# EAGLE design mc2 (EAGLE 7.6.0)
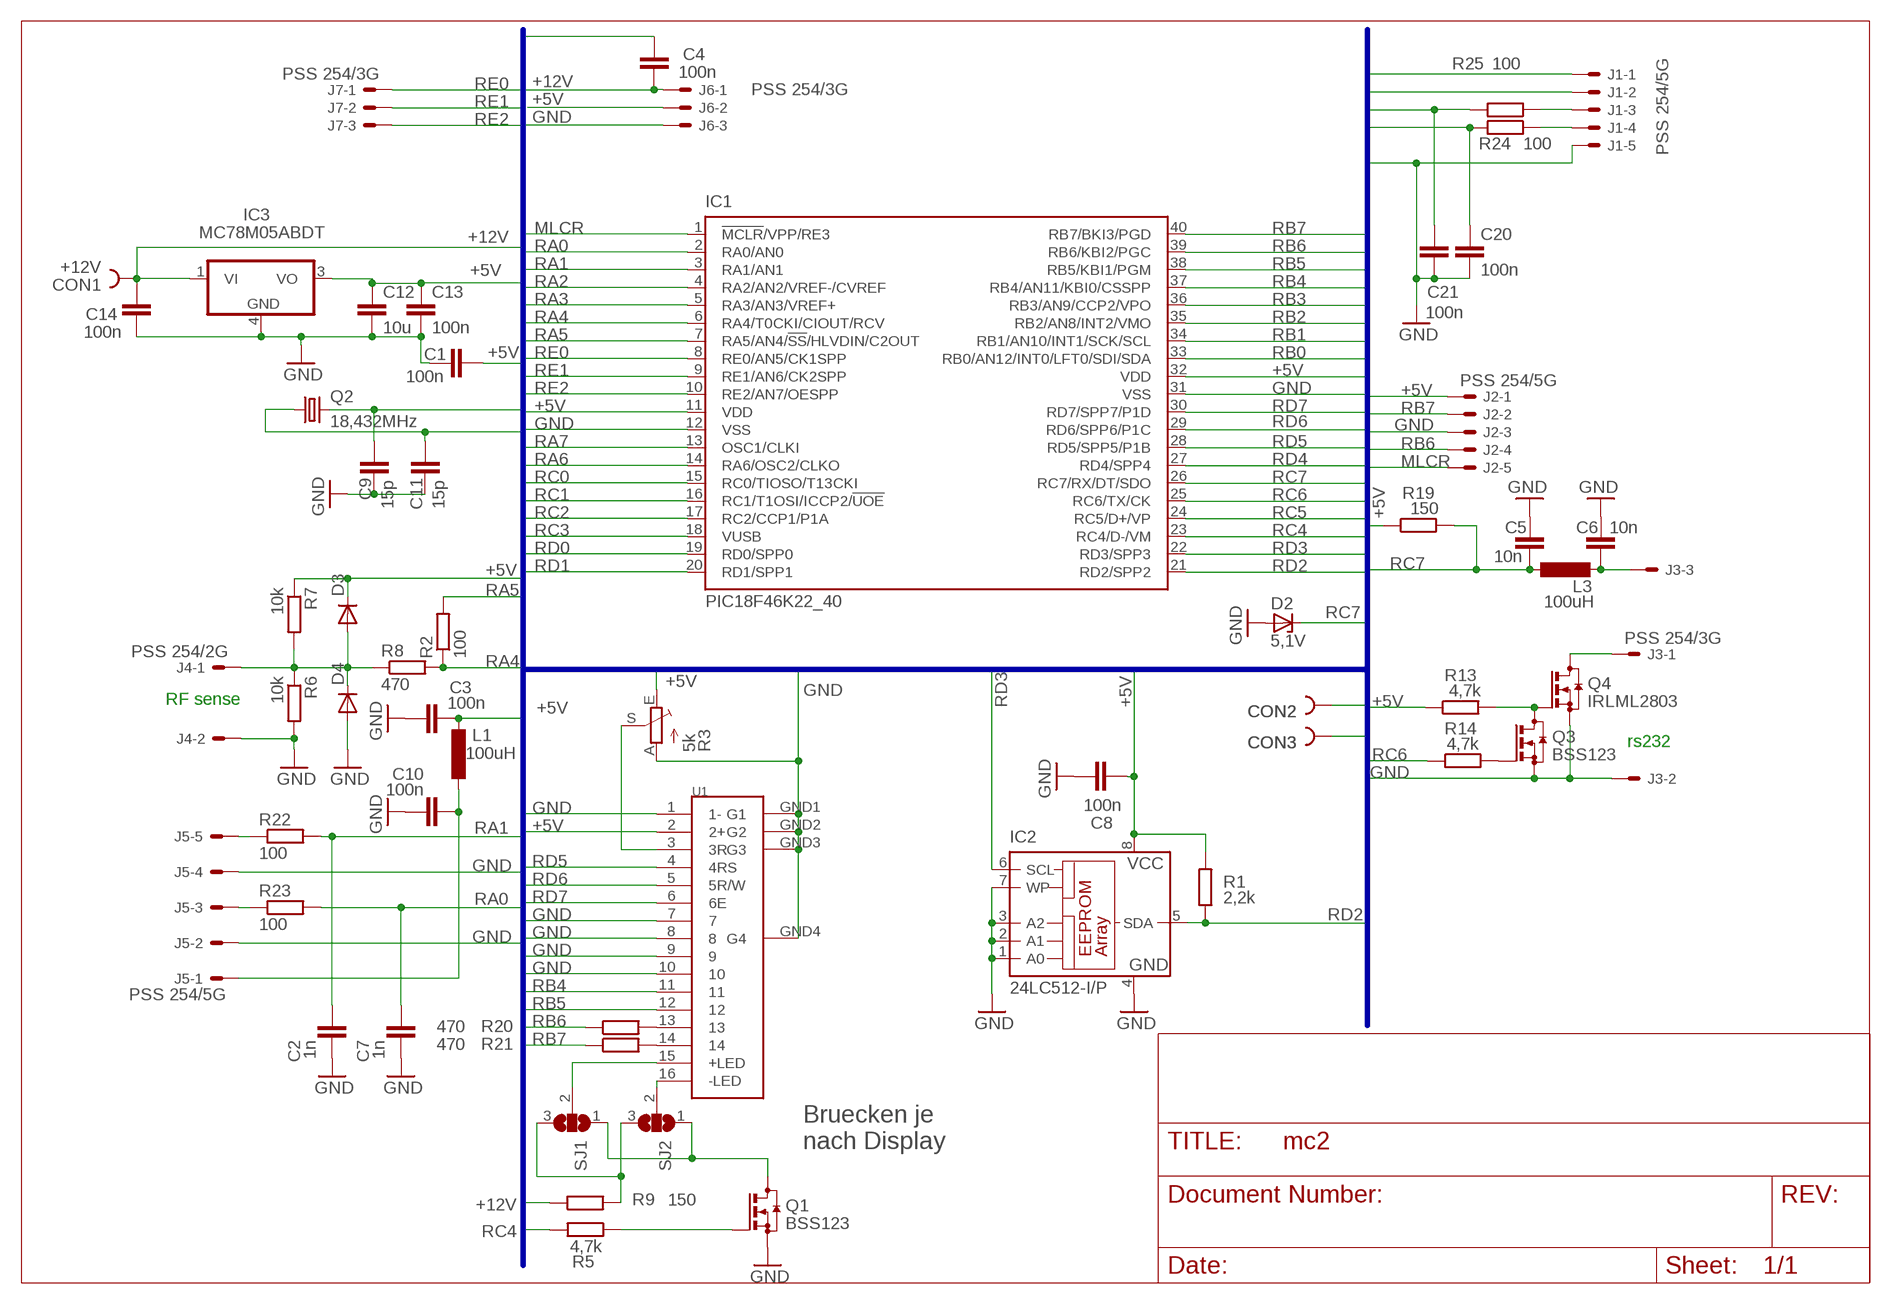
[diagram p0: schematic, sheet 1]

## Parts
C1  100n  C-EUC0805  [C0805]
C2  1n  C-EUC0805  [C0805]
C3  100n  C-EUC0805  [C0805]
C4  100n  C-EUC0805  [C0805]
C5  10n  C-EUC0805  [C0805]
C6  10n  C-EUC0805  [C0805]
C7  1n  C-EUC0805  [C0805]
C8  100n  C-EUC0805  [C0805]
C9  15p  C-EUC0805  [C0805]
C10  100n  C-EUC0805  [C0805]
C11  15p  C-EUC0805  [C0805]
C12  10u  C-EUC1206K  [C1206K]
C13  100n  C-EUC0805  [C0805]
C14  100n  C-EUC0805  [C0805]
C20  100n  C-EUC0805  [C0805]
C21  100n  C-EUC0805  [C0805]
CON1  +12V  PIN2_5  [PIN2_5]
CON2  PIN2_53MM  [HOLE3]
CON3  PIN2_53MM  [HOLE3]
D2  5,1V  ZENER-DIODESOT23  [SOT23]
D3  DIODE-SOD323-W  [SOD323-W]
D4  DIODE-SOD323-W  [SOD323-W]
IC1  PIC18F46K22_40  PIC18F4550_40  [DIL40]
IC2  24LC512-I/P  24AA32AP  [DIL8]
IC3  MC78M05ABDT  [DPACK_3]
J1  PSS 254/5G  22-27-2051-05  [6410-05]
J2  PSS 254/5G  22-27-2051-05  [6410-05]
J3  PSS 254/3G  22-27-2031-03  [6410-03]
J4  PSS 254/2G  22-27-2021-02  [6410-02]
J5  PSS 254/5G  22-27-2051-05  [6410-05]
J6  PSS 254/3G  22-27-2031-03  [6410-03]
J7  PSS 254/3G  22-27-2031-03  [6410-03]
L1  100uH  L-EUL2825P  [L2825P]
L3  100uH  L-EUL2825P  [L2825P]
Q1  BSS123  [SOT23]
Q2  18,432MHz  CRYSTALHC49U-V  [HC49U-V]
Q3  BSS123  [SOT23]
Q4  IRLML2803  BSS123  [SOT23]
R1  2,2k  R-EU_M0805  [M0805]
R2  100  R-EU_M0805  [M0805]
R3  5k  TRIM_EU-CA6V  [CA6V]
R5  4,7k  R-EU_M0805  [M0805]
R6  10k  R-EU_M0805  [M0805]
R7  10k  R-EU_M0805  [M0805]
R8  470  R-EU_M0805  [M0805]
R9  150  R-EU_0309/10  [0309/10]
R13  4,7k  R-EU_M0805  [M0805]
R14  4,7k  R-EU_M0805  [M0805]
R19  150  R-EU_M0805  [M0805]
R20  470  R-EU_M0805  [M0805]
R21  470  R-EU_M0805  [M0805]
R22  100  R-EU_M0805  [M0805]
R23  100  R-EU_M0805  [M0805]
R24  100  R-EU_M0805  [M0805]
R25  100  R-EU_M0805  [M0805]
SJ1  SJ2W  [SJ_2]
SJ2  SJ2W  [SJ_2]
U1  LCD_DOTOBEN  [LCD2X16_1]

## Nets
+5V: C1.1 C3.2 C8.1 C12.1 C13.1 D3.C IC1.11(VDD) IC1.32(VDD) IC2.8(VCC) IC3.3(VO) J2.1 J6.2 L1.2 R1.2 R3.E R7.1 R13.1 R19.1 U1.2(2+)
+12V: C4.2 C14.1 CON1.1 IC3.1(VI) J6.1 R9.1
GND: C1.2 C2.1 C3.1 C4.1 C5.1 C6.1 C7.1 C8.2 C9.2 C10.1 C11.2 C12.2 C13.2 C14.2 C20.2 C21.2 CON2.1 CON3.1 D2.1(A) D4.A IC1.12(VSS) IC1.31(VSS) IC2.1(A0) IC2.2(A1) IC2.3(A2) IC2.4(GND) IC2.7(WP) IC3.4(GND) J1.5 J2.3 J3.2 J4.2 J5.2 J5.4 J6.3 Q1.2(S) Q3.2(S) Q4.2(S) R3.A R6.2 U1.1(1-) U1.7 U1.8 U1.9 U1.10 U1.GND1(G1) U1.GND2(G2) U1.GND3(G3) U1.GND4(G4)
MLCR: IC1.1(!MCLR!/VPP/RE3) J2.5
N$1: R20.2 U1.13
N$2: R21.2 U1.14
N$3: R9.2 SJ1.3 SJ2.3
N$4: R3.S U1.3(3R)
N$5: SJ1.2 U1.15(+LED)
N$6: SJ2.2 U1.16(-LED)
N$7: Q1.1(G) R5.1
N$10: Q3.1(G) R14.2
N$11: J5.5 R22.1
N$12: C10.2 J5.1 L1.1
N$13: D3.A D4.C J4.1 R6.1 R7.2 R8.1
N$14: C6.2 J3.3 L3.2
N$15: J5.3 R23.1
N$16: J3.1 Q4.3(D)
N$17: Q1.3(D) SJ1.1 SJ2.1
N$36: Q3.3(D) Q4.1(G) R13.2
N$38: J1.4 R24.1
N$39: J1.3 R25.1
RA0: C7.2 IC1.2(RA0/AN0) R23.2
RA1: C2.2 IC1.3(RA1/AN1) R22.2
RA2: IC1.4(RA2/AN2/VREF-/CVREF)
RA3: IC1.5(RA3/AN3/VREF+)
RA4: IC1.6(RA4/T0CKI/CIOUT/RCV) R2.1 R8.2
RA5: IC1.7(RA5/AN4/!SS!/HLVDIN/C2OUT) R2.2
RA6: C9.1 IC1.14(RA6/OSC2/CLKO) Q2.2
RA7: C11.1 IC1.13(OSC1/CLKI) Q2.1
RB0: C20.1 IC1.33(RB0/AN12/INT0/LFT0/SDI/SDA) R24.2
RB1: C21.1 IC1.34(RB1/AN10/INT1/SCK/SCL) R25.2
RB2: IC1.35(RB2/AN8/INT2/VMO) J1.2
RB3: IC1.36(RB3/AN9/CCP2/VPO) J1.1
RB4: IC1.37(RB4/AN11/KBI0/CSSPP) U1.11
RB5: IC1.38(RB5/KBI1/PGM) U1.12
RB6: IC1.39(RB6/KBI2/PGC) J2.4 R20.1
RB7: IC1.40(RB7/BKI3/PGD) J2.2 R21.1
RC0: IC1.15(RC0/TIOSO/T13CKI)
RC1: IC1.16(RC1/T1OSI/ICCP2/!UOE)
RC2: IC1.17(RC2/CCP1/P1A)
RC3: IC1.18(VUSB)
RC4: IC1.23(RC4/D-/VM) R5.2
RC5: IC1.24(RC5/D+/VP)
RC6: IC1.25(RC6/TX/CK) R14.1
RC7: C5.2 D2.3(C) IC1.26(RC7/RX/DT/SDO) L3.1 R19.2
RD0: IC1.19(RD0/SPP0)
RD1: IC1.20(RD1/SPP1)
RD2: IC1.21(RD2/SPP2) IC2.5(SDA) R1.1
RD3: IC1.22(RD3/SPP3) IC2.6(SCL)
RD4: IC1.27(RD4/SPP4)
RD5: IC1.28(RD5/SPP5/P1B) U1.4(4RS)
RD6: IC1.29(RD6/SPP6/P1C) U1.5(5R/W)
RD7: IC1.30(RD7/SPP7/P1D) U1.6(6E)
RE0: IC1.8(RE0/AN5/CK1SPP) J7.1
RE1: IC1.9(RE1/AN6/CK2SPP) J7.2
RE2: IC1.10(RE2/AN7/OESPP) J7.3

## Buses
+12V,+5V,GND,RA[0..7],RB[0..7],RC[0..7],RD[0..7],RE[0..2],MLCR

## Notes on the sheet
- RF sense
- rs232
- Bruecken je 
  nach Display

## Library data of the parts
C1-C14 C20 C21 = rcl:C-EU: CAPACITOR, European symbol
CON1-CON3 = lindenau:PIN2_5
D2 = diode:ZENER-DIODE: Z-Diode
D3 D4 = diode:DIODE-: DIODE
IC1 = microchip:PIC18F4*_40: USB Microcontrollers with nanoWatt Technology High-Performance, Enhanced Flash, 28/40/44-Pin, Source: http://ww1.microchip.com/downloads/en/devicedoc/39632c.pdf
IC2 = microchip:24*: Serial EEPROM I2C
IC3 = linear:MC78M: 500 mA Positive Voltage Regulators Source: Data sheet
J1 J2 J5 = con-molex:22-?-05: CONNECTOR wire to board 2.54 mm (.1 inch) pitch header; OC_FARNELL: unknown; OC_NEWARK: unknown
J3 J6 J7 = con-molex:22-?-03: CONNECTOR wire to board 2.54 mm (.1 inch) pitch header; OC_FARNELL: unknown; OC_NEWARK: unknown
J4 = con-molex:22-?-02: CONNECTOR; OC_FARNELL: unknown; OC_NEWARK: unknown
L1 L3 = rcl:L-EU: INDUCTOR, European symbol
Q1 Q3 Q4 = transistor-small-signal:BSS123: N-CHANNEL MOS FET
Q2 = crystal:CRYSTAL: CRYSTAL; OC_FARNELL: 1666969; OC_NEWARK: unknown
R1 R2 R5-R9 R13 R14 R19-R25 = rcl:R-EU_: RESISTOR, European symbol
R3 = pot:TRIM_EU-: POTENTIOMETER
SJ1 SJ2 = jumper:SJ2W: SMD solder JUMPER
U1 = lindenau:LCD_DOT

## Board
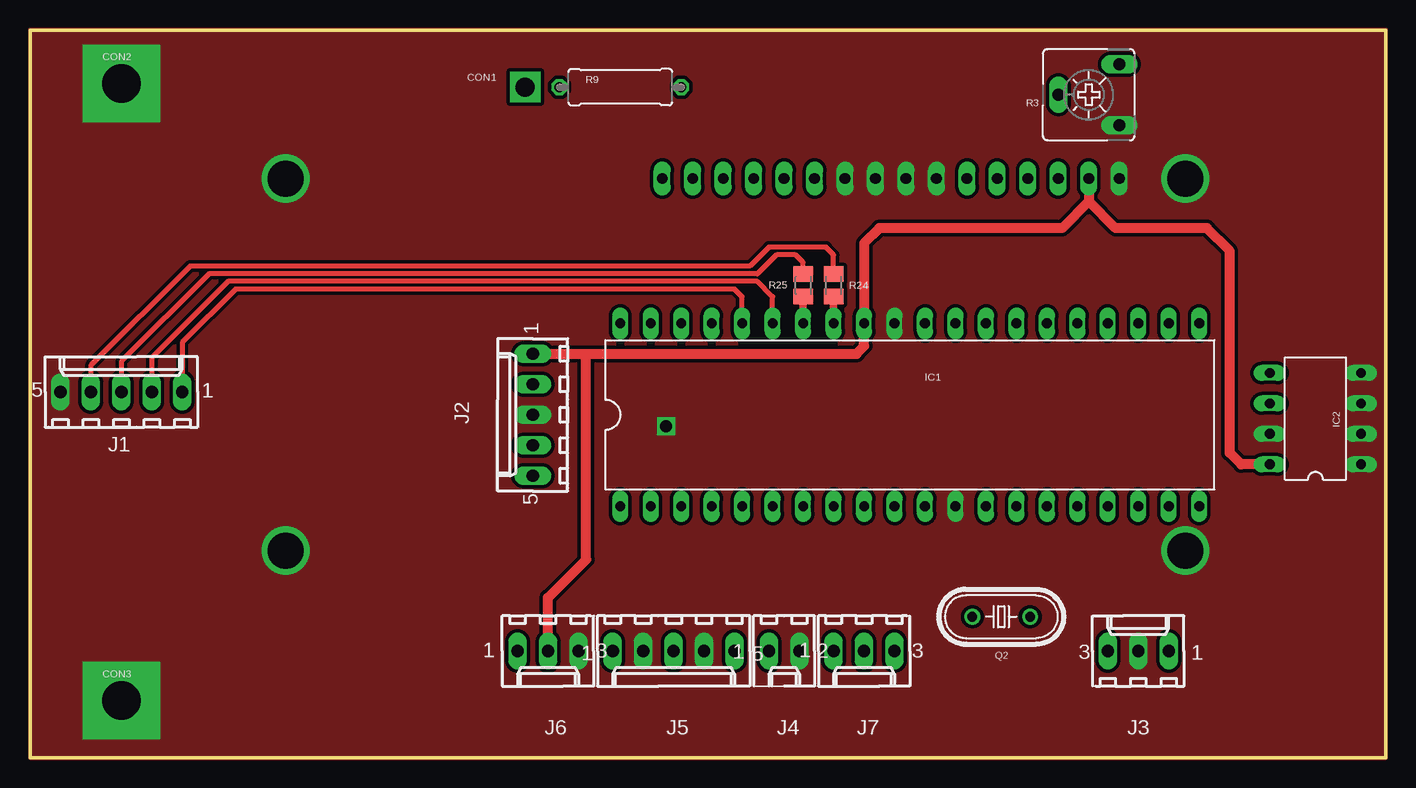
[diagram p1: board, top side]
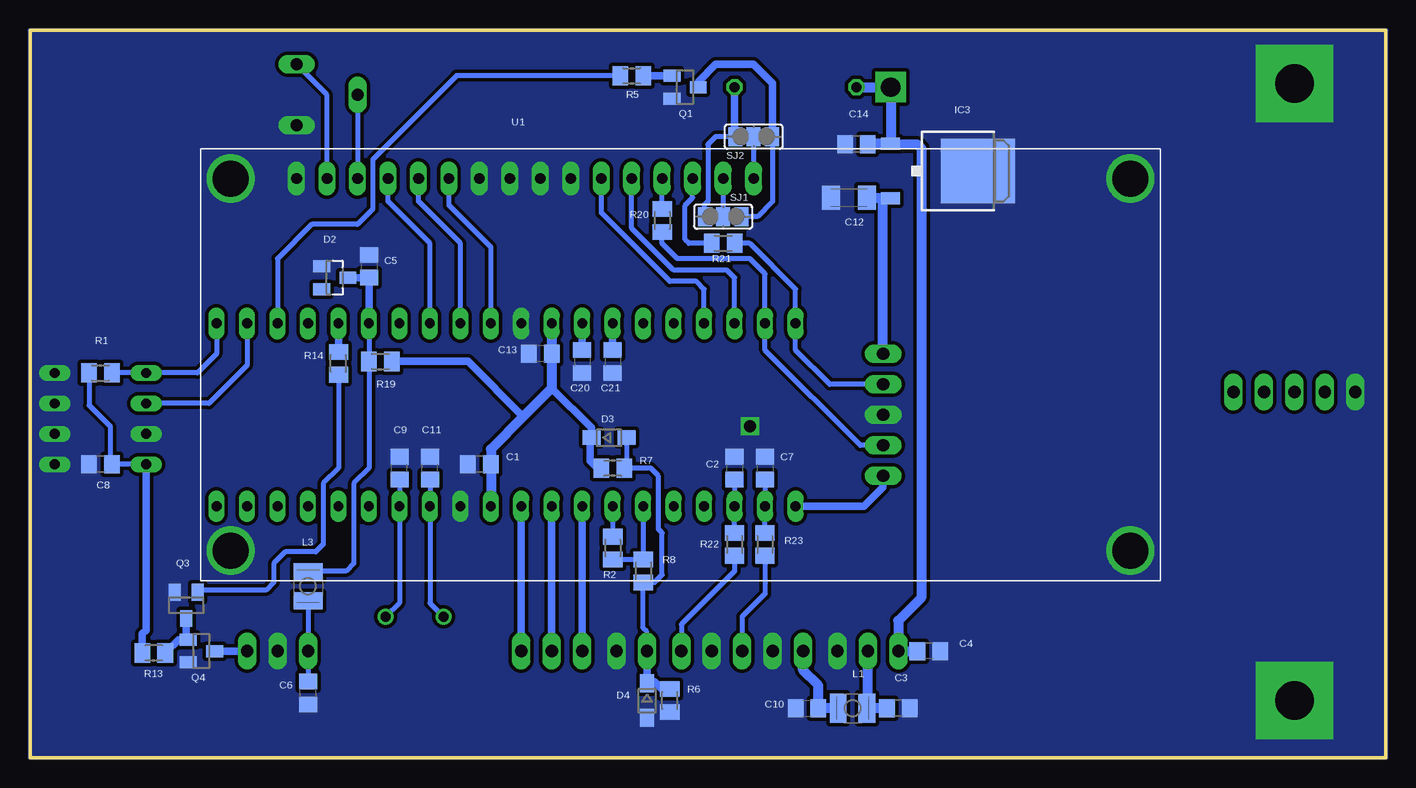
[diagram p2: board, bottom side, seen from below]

Size 113.03 x 60.64 mm. Coordinates in mm from the lower left corner, seen from the top.
Outline: 0,60.64 0,0 113.03,0 113.03,60.64 0,60.64
Copper layers (1*16): Top 0.035mm / dielectric 1.5mm / Bottom 0.035mm
Design rules "default *": minimum track width 10mil, minimum drill 24mil, track to track 8mil, track to pad 8mil, pad to pad 8mil, via to via 8mil, smd to smd 8mil, copper to edge 0mil, drill to drill 8mil, minimum pad ring 10mil, minimum via ring 8mil, stop-mask expansion 4mil, vias tented up to drill 0mil, thermal gap 10mil

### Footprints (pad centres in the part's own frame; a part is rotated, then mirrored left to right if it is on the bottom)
C0805 = smd 1.3 x 1.5: 1 -0.95,0; 2 0.95,0
C1206K = smd 1.5 x 2: 1 -1.5,0; 2 1.5,0
PIN2_5 = drill 1.6 pad 2.54 square: 1 0,0
HOLE3 = drill 3.2 pad 6.452 square: 1 0,0
SOT23 = smd 1 x 1.4: 1 -0.95,-1.1; 2 0.95,-1.1; 3 0,1.1
SOD323-W = smd 1.5 x 1.2: A 1.45,0; C -1.45,0
DIL40 = drill 0.813 long: 1 -24.13,-7.62; 2 -21.59,-7.62; 3 -19.05,-7.62; 4 -16.51,-7.62; 5 -13.97,-7.62; 6 -11.43,-7.62; 7 -8.89,-7.62; 8 -6.35,-7.62; 9 -3.81,-7.62; 10 -1.27,-7.62; 11 1.27,-7.62; 12 3.81,-7.62; 13 6.35,-7.62; 14 8.89,-7.62; 15 11.43,-7.62; 16 13.97,-7.62; 17 16.51,-7.62; 18 19.05,-7.62; 19 21.59,-7.62; 20 24.13,-7.62; 21 24.13,7.62; 22 21.59,7.62; 23 19.05,7.62; 24 16.51,7.62; 25 13.97,7.62; 26 11.43,7.62; 27 8.89,7.62; 28 6.35,7.62; 29 3.81,7.62; 30 1.27,7.62; 31 -1.27,7.62; 32 -3.81,7.62; 33 -6.35,7.62; 34 -8.89,7.62; 35 -11.43,7.62; 36 -13.97,7.62; 37 -16.51,7.62; 38 -19.05,7.62; 39 -21.59,7.62; 40 -24.13,7.62
DIL8 = drill 0.813 long: 1 -3.81,-3.81; 2 -1.27,-3.81; 3 1.27,-3.81; 4 3.81,-3.81; 5 3.81,3.81; 6 1.27,3.81; 7 -1.27,3.81; 8 -3.81,3.81
DPACK_3 = smd 1 x 1.6: 1 -2.28,-4.8; 3 2.28,-4.8 | smd 5.4 x 6.2: 4 0,2.5
6410-05 = drill 1.016 long: 1 5.08,0; 2 2.54,0; 3 0,0; 4 -2.54,0; 5 -5.08,0
6410-03 = drill 1.016 long: 1 2.54,0; 2 0,0; 3 -2.54,0
6410-02 = drill 1.016 long: 1 1.27,0; 2 -1.27,0
L2825P = smd 1.4 x 2.4: 1 -1.2,0; 2 1.2,0
HC49U-V = drill 0.813: 1 -2.413,0; 2 2.413,0
M0805 = smd 1.3 x 1.6: 1 -0.95,0; 2 0.95,0
CA6V = drill 1.016 long: A -2.54,-2.54; E 2.54,-2.54; S 0,2.54
0309/10 = drill 0.813 octagon: 1 -5.08,0; 2 5.08,0
SJ_2 = smd 1.168 x 1.6: 1 -1.524,0; 2 0,0; 3 1.524,0
LCD2X16_1 = drill 0.9 long: 1 5.397,0; 2 7.938,0; 3 10.477,0; 4 13.018,0; 5 15.557,0; 6 18.098,0; 7 20.637,0; 8 23.177,0; 9 25.718,0; 10 28.258,0; 11 30.797,0; 12 33.337,0; 13 35.877,0; 14 38.417,0; 15 40.958,0; 16 43.498,0 | drill 3: GND1 -0.102,0; GND2 74.897,0; GND3 74.897,-31; GND4 -0.102,-31

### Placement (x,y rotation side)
C1  75.56,24.45 180 bottom
C2  54.29,24.13 270 bottom
C3  40.64,4.13 180 bottom
C4  38.1,8.89 180 bottom
C5  84.77,40.96 270 bottom
C6  89.85,5.4 90 bottom
C7  51.75,24.13 270 bottom
C8  107.16,24.45 180 bottom
C9  82.23,24.13 90 bottom
C10  48.26,4.13 0 bottom
C11  79.69,24.13 90 bottom
C12  44.77,46.67 180 bottom
C13  70.48,33.66 180 bottom
C14  44.13,51.12 180 bottom
C20  66.99,33.02 270 bottom
C21  64.45,33.02 270 bottom
CON1  41.27,55.88 0 top
CON2  7.62,56.2 0 top
CON3  7.62,4.76 0 top
D2  87.63,40.01 270 bottom
D3  64.77,26.67 0 bottom
D4  61.59,4.76 270 bottom
IC1  73.34,28.57 0 top
IC2  107.16,28.26 90 top
IC3  36.51,48.9 270 bottom
J1  7.62,30.48 0 top
J2  41.91,28.57 90 top
J3  92.39,8.89 0 top
J4  62.87,8.89 180 top
J5  53.66,8.89 180 top
J6  43.18,8.89 180 top
J7  69.53,8.89 180 top
L1  44.45,4.13 0 bottom
L3  89.85,14.29 270 bottom
Q1  58.42,55.88 270 bottom
Q2  80.96,11.75 0 top
Q3  100.01,12.7 180 bottom
Q4  98.74,8.89 270 bottom
R1  107.16,32.07 180 bottom
R2  64.45,17.46 90 bottom
R3  88.27,55.24 90 top
R5  62.87,56.83 180 bottom
R6  59.69,4.76 270 bottom
R7  64.45,24.13 0 bottom
R8  61.91,15.56 90 bottom
R9  49.21,55.88 0 top
R13  102.71,8.73 0 bottom
R14  87.31,32.86 270 bottom
R19  83.82,33.02 180 bottom
R20  60.33,44.77 90 bottom
R21  55.24,42.86 180 bottom
R22  54.29,17.78 90 bottom
R23  51.75,17.78 90 bottom
R24  66.99,39.37 270 top
R25  64.45,39.37 270 top
SJ1  55.24,45.09 180 bottom
SJ2  52.7,51.75 180 bottom
U1  96.2,48.26 0 bottom

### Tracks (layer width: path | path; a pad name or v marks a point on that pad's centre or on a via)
+5V
  Top 0.813: U1.2 88.27,46.35 | 88.27,46.35 86.04,44.13 70.8,44.13 69.53,42.86 IC1.32 69.53,34.29 68.9,33.66 46.35,33.66 | IC2.8 100.97,24.45 100.01,25.4 100.01,42.23 98.11,44.13 90.49,44.13 88.27,46.35 | J2.1 46.35,33.66 | J6.2 43.18,13.34 46.35,16.51 46.35,33.66
  Bottom 0.406: R1.2 108.11,29.37 106.36,27.62 106.36,24.6 C8.1 IC2.8 | U1.2 88.27,55.24 R3.E
  Bottom 0.61: 71.91,28.42 76.52,33.02 R19.1 | R7.1 65.72,24.13 66.36,24.77 66.36,26.53 D3.C 66.22,27.48 69.53,30.8 | IC2.8 103.35,10.64 103.66,10.32 R13.1
  Bottom 0.813: IC3.3 41.91,46.62 | 41.91,46.62 43.21,46.62 C12.1 | C1.1 74.61,25.72 71.91,28.42 69.53,30.8 C13.1 IC1.32 | C1.1 | C1.1 IC1.11 | J2.1 41.91,46.62 | J6.2 43.18,4.13 L1.2 C3.2
+12V
  Bottom 0.813: R9.1 CON1.1 41.27,51.21 IC3.1 43.12,51.17 C14.1 39.05,51.12 38.73,50.8 38.73,13.34 40.64,11.43 J6.1 C4.2
GND  (via drill 1)
  other vias: 53.02,27.62
  pour Bottom (isolate 0.305, no thermals): 0,60.64 0,0 113.03,0 113.03,60.64
  pour Top (isolate 0.305, no thermals): 0,60.64 0,0 113.03,0 113.03,60.64
MLCR
  Bottom 0.61: J2.5 41.91,22.54 43.5,20.95 IC1.1
N$1
  Bottom 0.406: R20.2 U1.13
N$2
  Bottom 0.406: R21.2 58.1,42.86 58.42,43.18 58.42,46.04 57.78,46.67 U1.14
N$3
  Bottom 0.406: SJ2.3 55.88,51.75 56.52,51.12 56.52,46.35 56.83,46.04 56.83,45.15 SJ1.3
  Bottom 0.61: R9.2 54.29,51.82 SJ2.3
N$4
  Bottom 0.406: R3.S U1.3
N$5
  Bottom 0.406: U1.15 SJ1.2
N$6
  Bottom 0.406: SJ2.2 U1.16
N$7
  Bottom 0.61: Q1.1 R5.1
N$10
  Bottom 0.406: R14.2 87.31,24.13 88.58,22.86 88.58,17.78 89.22,17.14 91.76,17.14 92.71,16.19 92.71,14.61 93.34,13.97 98.89,13.97 Q3.1
N$11
  Bottom 0.406: R22.1 54.29,15.56 58.74,11.11 J5.5
N$12
  Bottom 0.813: L1.1 C10.2 47.31,6.04 48.58,7.3 J5.1
N$13
  Bottom 0.406: D3.A 63.32,24.31 R7.2 61.28,24.13 60.64,23.5 60.64,19.05 60.33,18.73 60.33,15.24 60.96,14.61 R8.1 61.91,10.79 61.59,10.48 J4.1
  Bottom 0.61: J4.1 D4.C 61.46,6.35 60.96,6.35 60.32,5.71 R6.1
N$14
  Bottom 0.406: L3.2 J3.3 C6.2
N$15
  Bottom 0.406: R23.1 51.75,13.65 53.66,11.75 J5.3
N$16
  Bottom 0.61: J3.1 Q4.3
N$17
  Bottom 0.406: SJ2.1 51.12,51.75 51.12,46.35 52.39,45.09 SJ1.1
  Bottom 0.61: Q1.3 57.32,56.34 55.88,57.78 52.7,57.78 51.12,56.2 51.12,51.82 SJ2.1
N$36
  Bottom 0.61: Q3.3 100.01,10.01 Q4.1 100.65,9.84 R13.2
N$38
  Top 0.406: R24.1 66.99,41.91 66.36,42.55 61.59,42.55 60.01,40.96 13.34,40.96 5.08,32.7 J1.4
N$39
  Top 0.406: R25.1 64.45,41.27 63.82,41.91 62.23,41.91 60.64,40.32 14.92,40.32 7.62,33.02 J1.3
RA0
  Bottom 0.406: R23.2 IC1.2 C7.2
RA1
  Bottom 0.406: R22.2 IC1.3 C2.2
RA4
  Bottom 0.406: R2.1 R8.2 IC1.6
RA5
  Bottom 0.406: IC1.7 R2.2
RA6
  Bottom 0.406: Q2.2 82.23,12.89 IC1.14 C9.1
RA7
  Bottom 0.406: Q2.1 79.69,12.89 IC1.13 C11.1
RB0
  Top 0.61: R24.2 IC1.33
  Bottom 0.61: IC1.33 C20.1
RB1
  Top 0.61: R25.2 IC1.34
  Bottom 0.61: IC1.34 C21.1
RB2
  Top 0.406: IC1.35 61.91,38.42 60.64,39.69 16.51,39.69 10.16,33.34 J1.2
RB3
  Top 0.406: IC1.36 59.37,38.42 58.74,39.05 17.14,39.05 12.7,34.61 J1.1
RB4
  Bottom 0.406: IC1.37 56.83,39.05 57.47,39.69 59.69,39.69 65.41,45.4 U1.11
RB5
  Bottom 0.406: IC1.38 54.29,40.01 54.93,40.64 59.37,40.64 62.87,44.13 U1.12
RB6
  Bottom 0.406: R20.1 60.33,42.86 59.05,41.59 53.02,41.59 51.75,40.32 IC1.39 51.75,33.97 43.81,26.04 J2.4
RB7
  Bottom 0.406: R21.1 53.02,42.86 49.21,39.05 IC1.40 49.21,33.97 46.35,31.11 J2.2
RC4
  Bottom 0.406: R5.2 77.47,56.83 84.45,49.85 84.45,45.72 85.72,44.45 89.53,44.45 92.39,41.59 IC1.23
RC6
  Bottom 0.61: IC1.25 R14.1
RC7
  Bottom 0.406: L3.1 89.78,15.56 86.68,15.56 86.04,16.19 86.04,22.86 84.77,24.13 R19.2 IC1.26
  Bottom 0.61: IC1.26 C5.2 D2.3
RD2
  Bottom 0.406: IC1.21 97.47,33.66 99.06,32.07 IC2.5 R1.1
RD3
  Bottom 0.406: IC1.22 94.93,32.7 98.11,29.53 IC2.6
RD5
  Bottom 0.406: IC1.28 79.69,42.86 83.19,46.35 U1.4
RD6
  Bottom 0.406: IC1.29 77.15,42.86 80.64,46.35 U1.5
RD7
  Bottom 0.406: IC1.30 74.61,42.55 78.11,46.04 U1.6
RE0
  Bottom 0.61: IC1.8 J7.1
RE1
  Bottom 0.61: IC1.9 J7.2
RE2
  Bottom 0.61: IC1.10 J7.3

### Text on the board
Document: Dreh_Taste | Programmer | SV Relaisdriver | Messkopf | Frq-mess | RelaisDriver | rs232
tDocu: 12V | 5V | GND | 5V | GND | Uvor | GND | Urueck | CLK | Cdata | Latch | RX | GND | TX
